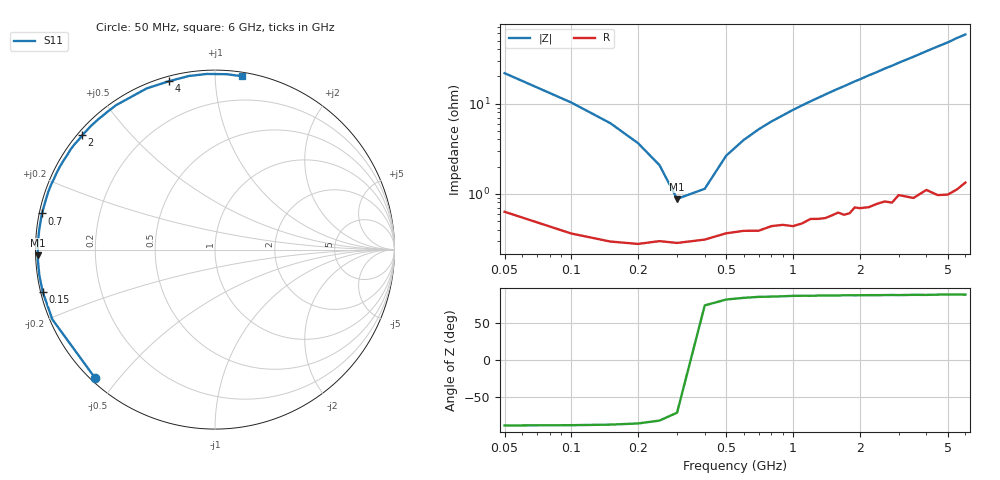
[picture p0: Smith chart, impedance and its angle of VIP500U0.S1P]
! Infineon Technologies  Discrete & RF Semiconductors
! BB 804
! Si Tuning Diode in SOT23
! VR = 0.5 V
! S-Parameters:  July  1999
# GHz  S  MA  R  50
!  f  S11
! GHz  MAG  ANG
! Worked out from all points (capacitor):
!   34 points, 50 MHz to 6 GHz, reference 50 ohm
!   read as one part to ground: C = 142 pF near 50 MHz
!   lowest |Z| = 876 mohm at 300 MHz (marker M1)
!   series resonance near 343.2 MHz, so ESL is about 1.5 nH
!   S11 on the Smith chart (normalised r, x): 50 MHz: 0.01, -0.43; 150 MHz: 0.01, -0.12; 700 MHz: 0.01, +0.10; 2 GHz: 0.01, +0.37; 4 GHz: 0.02, +0.76; 6 GHz: 0.03, +1.17
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0.05  0.979 -133.0
0.1  0.9862 -156.8
0.15  0.9885 -166.2
0.2  0.989 -171.7
0.25  0.9882 -175.3
0.3  0.9887 -178.1
0.4  0.9877 177.5
0.5  0.9856 174.0
0.7  0.9848 168.2
0.8  0.9829 165.6
1  0.9832 160.7
1.2  0.9801 156.1
1.4  0.98 151.7
1.6  0.9775 147.4
1.7  0.9789 145.4
1.8  0.9784 143.3
2  0.976 139.3
2.2  0.976 135.3
2.4  0.9746 131.7
2.6  0.9739 127.8
2.8  0.9753 124.5
3  0.9712 120.9
3.5  0.9754 113.0
4  0.9725 105.4
4.5  0.978 98.6
5  0.9798 92.6
5.5  0.9794 86.2
6  0.9778 81.1
